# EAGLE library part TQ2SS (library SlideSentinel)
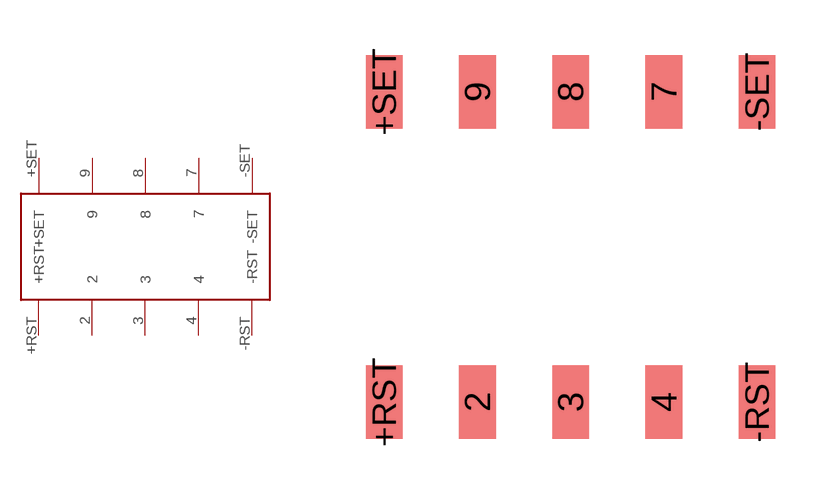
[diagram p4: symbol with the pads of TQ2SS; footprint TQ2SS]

Designator prefix -

## TQ2SS  [TQ2SS]
2  2
3  3
4  4
7  7
8  8
9  9
+RST  +RST
+SET  +SET
-RST  -RST
-SET  -SET

## Footprint TQ2SS (pad centres in mm)
smd 1 x 2: 2 -2.16,-4.418; 3 0.38,-4.418; 4 2.92,-4.418; 7 2.92,4.04; 8 0.38,4.04; 9 -2.16,4.04; +RST -4.7,-4.418; +SET -4.7,4.04; -RST 5.46,-4.418; -SET 5.46,4.04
